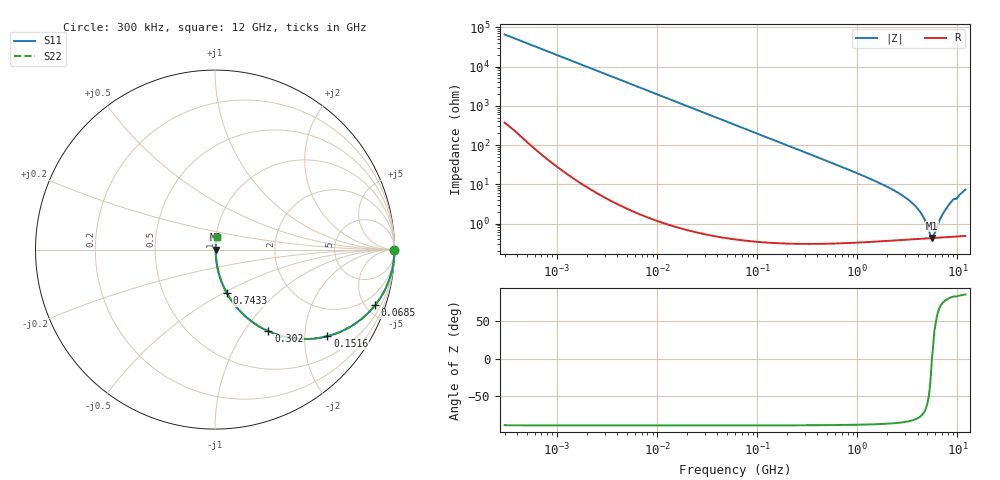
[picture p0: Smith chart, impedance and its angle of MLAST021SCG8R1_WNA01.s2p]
! MLAST021SCG8R1_WNA01  S-PARAMETER MODEL  ( General Type )
! Model Generated by TAIYO YUDEN Corporation (http://www.ty-top.com)
! Version 1.0
! TAIYO YUDEN Control No. 220901
! Copyright(c) 2022 TAIYO YUDEN CO.,LTD. All Rights Reserved.
! Product Description (link to TY-COMPAS)
! https://ds.yuden.co.jp/TYCOMPAS/or/detail?pn=MLAST021SCG8R1CWNA01&u=M
! Products Name : Multilayer Ceramic Capacitors
! Characteristics :
!  Capacitance : 8.1 pF , Rated Voltage : 25V , TCC : CG / C0G
!  Case Size : 0.25 x 0.125 / 0.0098 x 0.0049 [mm/inch] , Thickness : 0.125 / 0.0049 [mm/inch]
!  (Conditions: Temperature = 25 degC , DC Bias Current/Voltage = 0A / 0V)
! External Node Assignments :
!  1  o---| |---o  2
! GND o---------o GND
! Frequency Range : 0.3MHz  -  12000MHz  [ 401 STEP ]
# MHz S RI R 50
! Freq[MHz].  S11 Real  S11 Imag  S21 Real  S21 Imag  S12 Real  S12 Imag  S22 Real  S22 Imag
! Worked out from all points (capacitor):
!   401 points, 300 kHz to 12 GHz, reference 50 ohm
!   read as one part in series: C = 8.1 pF near 316.3 kHz
!   lowest |Z| = 428 mohm at 5.566 GHz (marker M1)
!   series resonance near 5.561 GHz, so ESL is about 100 pH
!   S11 on the Smith chart (normalised r, x): 300 kHz: open; 68.5 MHz: 1.01, -5.74; 151.6 MHz: 1.01, -2.59; 302 MHz: 1.01, -1.30; 743.3 MHz: 1.01, -0.52; 12 GHz: 1.01, +0.15
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0.3  1 -0.00153  1.1e-05 0.00153  1.1e-05 0.00153  1 -0.00153
1.769972  0.9999 -0.00901  8.94e-05 0.00901  8.94e-05 0.00901  0.9999 -0.00901
10.44266  0.9972 -0.053  0.00285 0.053  0.00285 0.053  0.9972 -0.053
27.10171  0.9812 -0.1353  0.0188 0.1353  0.0188 0.1353  0.9812 -0.1353
60  0.9144 -0.2792  0.0856 0.2792  0.0856 0.2792  0.9144 -0.2792
68.49786  0.8913 -0.3106  0.1087 0.3106  0.1087 0.3106  0.8913 -0.3106
101.9188  0.7875 -0.4082  0.2125 0.4082  0.2125 0.4082  0.7875 -0.4082
151.6462  0.6261 -0.4826  0.3739 0.4826  0.3739 0.4826  0.6261 -0.4826
301.9711  0.2971 -0.4547  0.7029 0.4547  0.7029 0.4547  0.2971 -0.4547
353.9943  0.2353 -0.4215  0.7647 0.4215  0.7647 0.4215  0.2353 -0.4215
743.2595  0.0657 -0.2418  0.9343 0.2418  0.9343 0.2418  0.0657 -0.2418
2088.533  0.01 -0.0797  0.99 0.0797  0.99 0.0797  0.01 -0.0797
3026.31  0.00591 -0.0452  0.9941 0.0452  0.9941 0.0452  0.00591 -0.0452
3841.137  0.00471 -0.0265  0.9953 0.0265  0.9953 0.0265  0.00471 -0.0265
4502.883  0.00434 -0.0149  0.9957 0.0149  0.9957 0.0149  0.00434 -0.0149
5278.635  0.00424 -0.00363  0.9958 0.00363  0.9958 0.00363  0.00424 -0.00363
5565.855  0.00426 6.58e-05  0.9957 -6.58e-05  0.9957 -6.58e-05  0.00426 6.58e-05
5868.704  0.00431 0.0032  0.9957 -0.0032  0.9957 -0.0032  0.00431 0.0032
6879.757  0.00461 0.0141  0.9954 -0.0141  0.9954 -0.0141  0.00461 0.0141
8064.993  0.00528 0.0275  0.9947 -0.0275  0.9947 -0.0275  0.00528 0.0275
8732.115  0.00584 0.0354  0.9942 -0.0354  0.9942 -0.0354  0.00584 0.0354
12000  0.0101 0.0722  0.9899 -0.0722  0.9899 -0.0722  0.0101 0.0722
